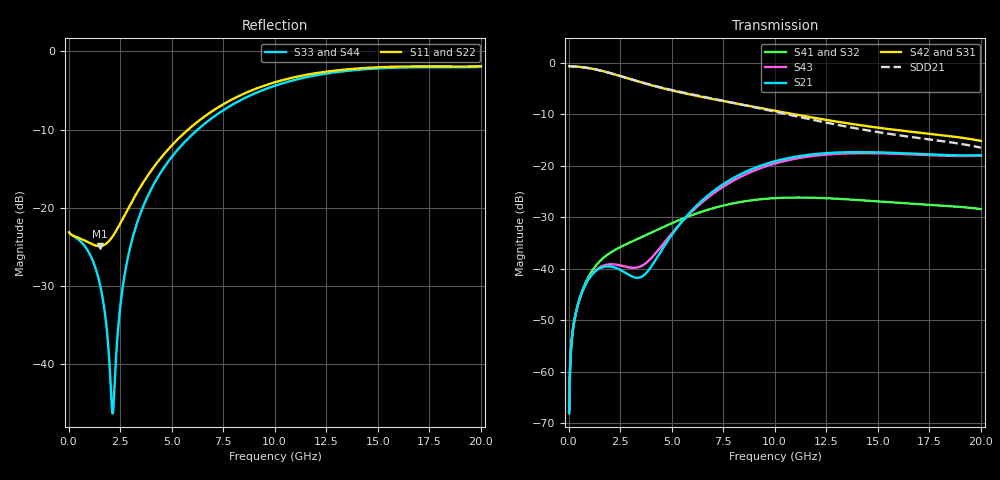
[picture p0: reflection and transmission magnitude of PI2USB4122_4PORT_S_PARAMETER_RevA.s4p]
! NPort=4 DATA=800 NOISE=0 GROUPDELAY=0 COMPLEX_DATAFORMAT=POLAR
! NumOfBlock=1 NumOfParam=0
! .MODEL Smodel S TSTONEFILE=PI2USB4122_4PORT_S_PARAMETER_RevA.s4p TYPE=S
!  -- The above .MODEL line can be used for the S element in the netlist.
! PORT DEFINITION
! PORT1 = INPUT+
! PORT2 = INPUT-
! PORT3 = OUTPUT+
! PORT4 = OUTPUT-
# Hz S MA R  50
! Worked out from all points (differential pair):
!   800 points, 25 MHz to 20 GHz, reference 50 ohm
!   strongest paths, dB at 25 MHz, 5.025 GHz, 10.03 GHz, 15.03 GHz, 20 GHz:
!     S42: -0.7, -5.4, -9.4, -12.6, -15.2
!     S31: -0.7, -5.4, -9.4, -12.6, -15.2
!     S21: -68.1, -33.4, -19.1, -17.4, -18.0
!     S43: -68.1, -33.1, -19.6, -17.6, -18.1
!     S41: -68.1, -31.2, -26.3, -26.9, -28.4
!     S32: -68.1, -31.2, -26.3, -26.9, -28.4
!   taken as a pair (ports 2,1 in; 4,3 out), SDD21 dB: -0.7, -5.3, -9.5, -13.5, -16.5
!   lowest |S11| = -24.9 dB at 1.5 GHz (marker M1), VSWR 1.12, Z = 48 - j5.19 ohm
!   |S11| at or under -10 dB: start of sweep to 5.803 GHz
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2.5e7  0.06952 -3.0  0.0003955 85.8  0.9245 -0.7  0.0003933 85.8
       0.0003955 85.8  0.06952 -3.0  0.0003933 85.8  0.9245 -0.7
       0.9245 -0.7  0.0003933 85.8  0.06956 -2.3  0.0003956 85.9
       0.0003933 85.8  0.9245 -0.7  0.0003956 85.9  0.06956 -2.3
4e8  0.06471 -26.2  0.004073 65.7  0.9147 -9.4  0.004087 65.1
     0.004073 65.7  0.06471 -26.2  0.004087 65.1  0.9147 -9.4
     0.9147 -9.4  0.004087 65.1  0.06347 -13.9  0.00407 66.4
     0.004087 65.1  0.9147 -9.4  0.00407 66.4  0.06347 -13.9
1.5e9  0.05666 -108.1  0.01004 51.7  0.8439 -33.8  0.0117 48.5
       0.01004 51.7  0.05666 -108.1  0.0117 48.5  0.8439 -33.8
       0.8439 -33.8  0.0117 48.5  0.03313 -51.8  0.01025 55.0
       0.0117 48.5  0.8439 -33.8  0.01025 55.0  0.03313 -51.8
2.15e9  0.06589 -165.4  0.01036 46.5  0.7788 -46.6  0.01478 38.6
        0.01036 46.5  0.06589 -165.4  0.01478 38.6  0.7788 -46.6
        0.7789 -46.6  0.01478 38.6  0.004819 -162.4  0.01101 51.4
        0.01478 38.6  0.7789 -46.6  0.01101 51.4  0.004819 -162.4
3.25e9  0.1203 124.8  0.008163 66.8  0.6678 -64.8  0.01903 27.1
        0.008163 66.8  0.1203 124.8  0.01903 27.1  0.6678 -64.8
        0.6678 -64.8  0.01903 27.1  0.07447 89.1  0.0102 68.5
        0.01903 27.1  0.6678 -64.8  0.0102 68.5  0.07447 89.1
6.175e9  0.3477 35.8  0.04028 113.9  0.4781 -102.0  0.03411 -6.1
         0.04028 113.9  0.3477 35.8  0.03411 -6.1  0.4781 -102.0
         0.4781 -101.9  0.03412 -6.1  0.3087 25.2  0.03895 106.8
         0.03412 -6.1  0.4781 -101.9  0.03895 106.8  0.3087 25.2
2e10  0.8046 -97.8  0.1261 5.3  0.1736 101.3  0.03786 146.5
      0.1261 5.3  0.8046 -97.8  0.03786 146.5  0.1736 101.3
      0.1737 101.3  0.03788 146.6  0.7965 -98.0  0.1247 5.9
      0.03788 146.6  0.1737 101.3  0.1247 5.9  0.7965 -98.0
